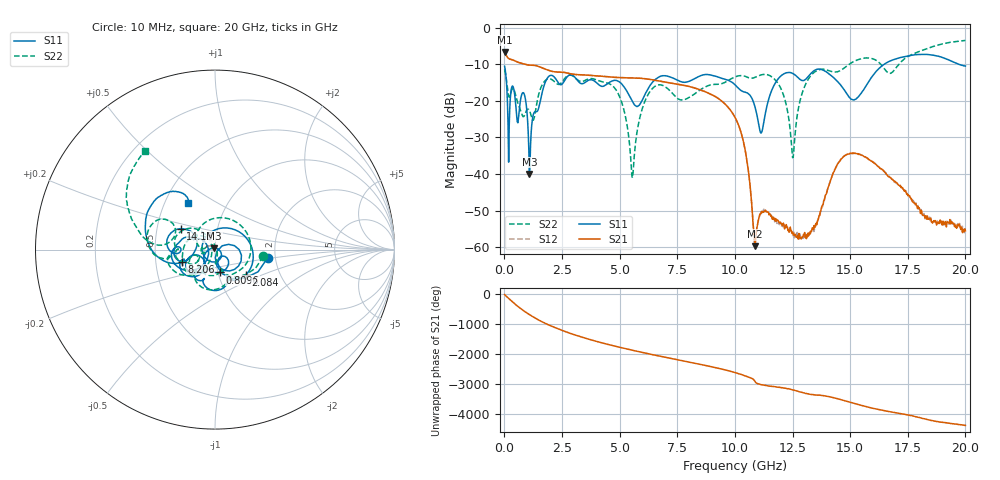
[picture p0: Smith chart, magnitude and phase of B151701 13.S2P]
!  2-Port S-parameters saved by WinCal
! VAR MeasName=S-Parameters (CALIBRATED_DATA) read from VNA (N5244A)
! VAR MeasDate=2015-12-24 19:09:38
! VAR NAME=B151701 13
! VAR FILENAME=B151701 13.S2P
! VAR DATE=2015-12-24 19:09:38
! VAR PHYS_PORTS=1,3
# Hz S DB R 50
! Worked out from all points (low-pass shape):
!   801 points, 10 MHz to 20 GHz, reference 50 ohm
!   highest |S21| = -6.63 dB at 10 MHz (marker M1); lowest = -59.7 dB at 10.88 GHz (marker M2)
!   |S21| within 3 dB of the highest: start of sweep to 704.1 MHz
!   lowest |S11| = -40.0 dB at 1.084 GHz (marker M3), VSWR 1.02, Z = 49.6 + j0.895 ohm
!   |S11| at or under -10 dB: start of sweep to 16.47 GHz; 19.72 GHz to end of sweep
!   |S22| runs from -41.1 to -3.5 dB; largest |S21 - S12| = 0.0021
!   S11 on the Smith chart (normalised r, x): 10 MHz: 1.82, -0.18; 809.6 MHz: 1.02, -0.26; 2.084 GHz: 1.34, -0.40; 8.206 GHz: 0.68, -0.09; 14.18 GHz: 0.66, +0.16; 20 GHz: 0.65, +0.37
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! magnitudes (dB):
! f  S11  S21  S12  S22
! 10 MHz  -10.5  -6.6  -6.6  -11.3
! 209.9 MHz  -26.8  -8.5  -8.5  -19.0
! 809.6 MHz  -17.7  -9.8  -9.8  -24.3
! 1.084 GHz  -40.0  -10.2  -10.2  -22.6
! 2.084 GHz  -13.1  -11.9  -11.9  -14.3
! 3.358 GHz  -15.3  -12.9  -12.9  -14.7
! 4.858 GHz  -14.4  -13.6  -13.6  -17.1
! 5.557 GHz  -20.2  -13.7  -13.7  -41.1
! 6.007 GHz  -19.5  -13.9  -13.9  -21.6
! 6.682 GHz  -13.5  -14.5  -14.5  -15.6
! 8.206 GHz  -14.1  -16.4  -16.4  -18.3
! 10.01 GHz  -15.6  -24.5  -24.5  -13.4
! 10.45 GHz  -17.6  -33.8  -33.8  -13.3
! 10.88 GHz  -21.8  -59.7  -58.9  -13.5
! 11.15 GHz  -28.7  -50.2  -50.3  -12.9
! 11.93 GHz  -13.6  -53.4  -53.8  -15.8
! 12.5 GHz  -12.5  -55.9  -56.8  -35.5
! 13.35 GHz  -12.1  -54.7  -55.1  -12.7
! 14.18 GHz  -13.0  -41.3  -41.2  -11.9
! 15.18 GHz  -19.7  -34.3  -34.3  -9.1
! 16.68 GHz  -9.2  -40.7  -40.7  -12.4
! 20 GHz  -10.5  -55.5  -55.3  -3.5
